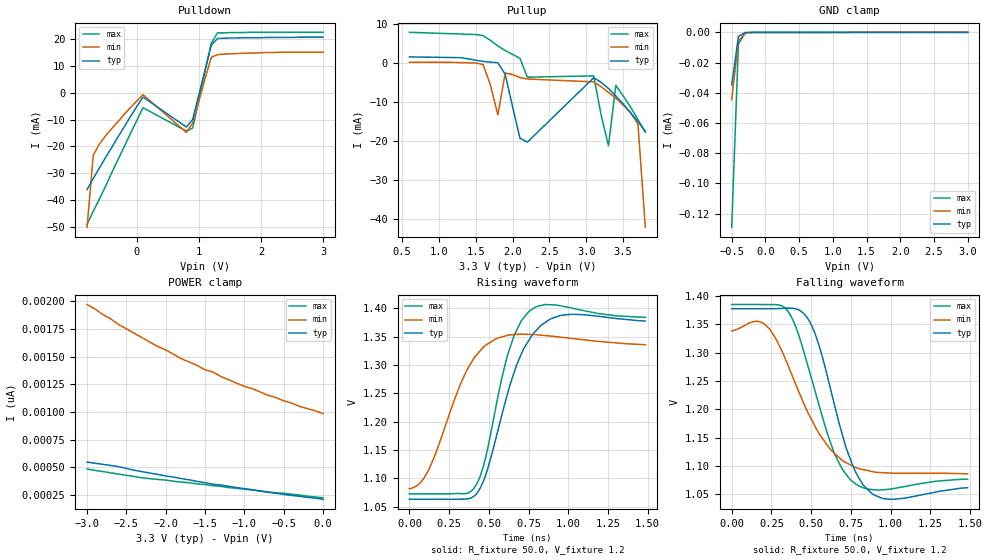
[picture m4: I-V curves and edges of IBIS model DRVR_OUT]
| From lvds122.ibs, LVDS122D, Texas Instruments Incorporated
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|   Driver Output Model
[Model]   DRVR_OUT
Model_type   Output
| Signals   1Y,1Z,2Y,2Z
Vmeas = 1.2V   |Reference voltage for timing measurements
Cref = 5pF   |Timing specification test load capacitance value
Rref = 50   |Note: 50 Ohm load; single ended configuration
| variable   typ   min   max
C_comp   2.5pF   1.9pF   3.0pF
|   typ   min   max
[Temperature Range]   25.0   85   -40
[Voltage range]   3.3V   3.0V   3.6V
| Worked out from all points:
|   rising waveform, R_fixture 50.0, V_fixture 1.2: 20-80 % time 195ps typ, 203ps min, 145ps max; typ from 1.06 V to 1.38 V
|   falling waveform, R_fixture 50.0, V_fixture 1.2: 20-80 % time 182ps typ, 262ps min, 195ps max; typ from 1.38 V to 1.06 V
[Pulldown]
|   Voltage   I(typ)   I(min)   I(max)
-800mV    -36mA      -50mA      -48.9mA
-700mV    -31.9mA    -23.2mA    -44.1mA
-600mV    -28mA      -19.1mA    -39.5mA
-500mV    -24mA      -16mA      -34.7mA
-200mV    -12.7mA    -8.01mA    -20mA
100mV     -1.64mA    -780uA     -5.62mA
800mV     -12.8mA    -14.8mA    -14.3mA
900mV     -9.98mA    -11.3mA    -13.2mA
1.2V      17.6mA     13.1mA     18.3mA
1.3V      20.1mA     14.1mA     22.2mA
2.1V      20.5mA     14.9mA     22.4mA
3V        20.6mA     15mA       22.4mA
[Pullup]
|   Voltage   I(typ)   I(min)   I(max)
| Note that the[Pullup]voltage table is referenced to Vcc
| and is calculated using Vtable=Vcc - Vmeasured.
600mV     1.67mA     314uA      7.97mA
1.6V      517uA      -293uA     7.12mA
1.8V      156uA      -13.2mA    4.48mA
1.9V      -2.8mA     -2.46mA    3.29mA
2.1V      -19.2mA    -3.64mA    1.3mA
2.2V      -20.2mA    -4mA       -3.53mA
3.1V      -3.68mA    -4.74mA    -3.2mA
3.2V      -4.85mA    -5.97mA    -13.2mA
3.3V      -6.42mA    -7.47mA    -21.1mA
3.4V      -8.34mA    -8.87mA    -5.62mA
3.7V      -14.9mA    -15.6mA    -14.4mA
3.8V      -17.5mA    -42mA      -17.6mA
[GND_clamp]
|   Voltage   I(typ)   I(min)   I(max)
| Outputs in High Impedance (off)
-500mV    -34.9uA    -44.4uA    -129uA
-400mV    -2.66uA    -5.59uA    -7.81uA
-300mV    -143nA     -725nA     -280nA
-100mV    -4.95nA    -142nA     -1.46nA
3V        185pA      984pA      178pA
[POWER_clamp]
|   Voltage   I(typ)   I(min)   I(max)
| Note that the [POWER_clamp] voltage table is referenced to Vcc
| and is calculated using Vtable = Vcc - Vmeasured.
| Outputs in Tri-state.
-3V       546pA      1.97nA     483pA
-2.9V     536pA      1.93nA     472pA
-2.6V     506pA      1.79nA     438pA
-2.3V     460pA      1.67nA     404pA
-2.1V     435pA      1.59nA     390pA
-1.8V     397pA      1.48nA     366pA
-1.5V     360pA      1.38nA     343pA
-1.4V     347pA      1.36nA     333pA
-1.3V     339pA      1.32nA     327pA
-700mV    274pA      1.15nA     277pA
-300mV    238pA      1.05nA     249pA
0V        210pA      984pA      224pA
[Ramp]
|   typ   min   max
dV/dt_r   0.20/206ps   0.20/287ps   0.20/154ps
dV/dt_f   0.20/194ps   0.20/358ps   0.20/228ps
R_load = 50ohm |Note: The measurement is on a single-ended configuration
|   with 100ohm line-to-line.
[Rising Waveform]
R_fixture = 50.0
V_fixture = 1.2
C_fixture = 0p
L_fixture = 0n
|   V(typ)   V(min)   V(max)
0s        1.063V     1.082V     1.072V
120ps     1.063V     1.114V     1.072V
390ps     1.065V     1.304V     1.077V
465ps     1.094V     1.331V     1.12V
540ps     1.165V     1.345V     1.22V
660ps     1.287V     1.353V     1.352V
750ps     1.343V     1.354V     1.394V
825ps     1.369V     1.353V     1.405V
1.02ns    1.389V     1.347V     1.401V
1.485ns   1.377V     1.336V     1.384V
[Falling Waveform]
R_fixture = 50.0
V_fixture = 1.2
C_fixture = 0p
L_fixture = 0n
|   V(typ)   V(min)   V(max)
0s        1.378V     1.338V     1.385V
150ps     1.378V     1.355V     1.385V
240ps     1.377V     1.341V     1.385V
360ps     1.379V     1.274V     1.371V
465ps     1.366V     1.203V     1.291V
540ps     1.321V     1.162V     1.217V
645ps     1.21V      1.123V     1.123V
780ps     1.089V     1.097V     1.068V
960ps     1.042V     1.088V     1.058V
1.485ns   1.062V     1.086V     1.076V
